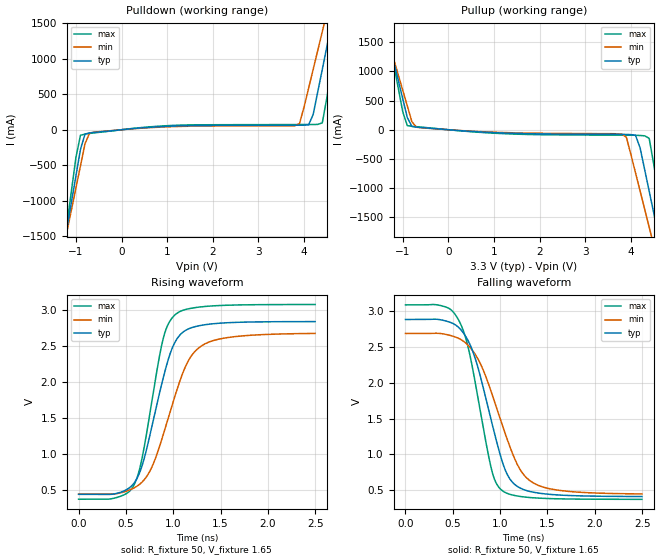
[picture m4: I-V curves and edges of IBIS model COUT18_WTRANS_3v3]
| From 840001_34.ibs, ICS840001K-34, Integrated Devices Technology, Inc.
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[Model] COUT18_WTRANS_3v3
Model_type   Output
Polarity   Non-Inverting
|   typ   min   max
C_comp   2pF   1.5pF   2.5pF
Vmeas = 1.65V
Rref = 50
Cref = 0
Vref = 1.65V
|   typ   min   max
[Voltage range]   3.3V   3.135V   3.465V
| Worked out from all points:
|   slope of the pulldown table from 0 to 0.495 V, typ, clamps not added: 17.2 ohm
|   slope of the pullup table from 0 to 0.495 V, typ, clamps not added: 17.5 ohm
|   rising waveform, R_fixture 50, V_fixture 1.65: 20-80 % time 269ps typ, 337ps min, 216ps max; typ from 0.443 V to 2.84 V
|   falling waveform, R_fixture 50, V_fixture 1.65: 20-80 % time 296ps typ, 367ps min, 235ps max; typ from 2.88 V to 0.414 V
[Pulldown]
|Voltage   I (typ)   I (min)   I (max)
-3.3V     -9.29A     -8.033A    -11.4A
-1.3V     -1.781A    -1.764A    -1.832A
-1.2V     -1.405A    -1.45A     -1.352A
-900mV    -277.4mA   -509.6mA   -77.59mA
-800mV    -60.69mA   -196.4mA   -61.25mA
-600mV    -38.28mA   -33.91mA   -44.11mA
3.9V      63.76mA    86.74mA    73.17mA
4.2V      215.8mA    852.4mA    74.01mA
4.4V      853.2mA    1.385A     97.44mA
4.6V      1.492A     1.918A     860.7mA
4.8V      2.133A     2.453A     1.678A
6.6V      8.005A     7.35A      9.166A
[Pullup]
|Voltage   I (typ)   I (min)   I (max)
-3.3V     7.952A     6.873A     9.764A
-1.4V     1.821A     1.753A     1.953A
-900mV    207mA      406.2mA    70.87mA
-700mV    45.36mA    43.45mA    52.59mA
3.8V      -79.73mA   -73.83mA   -93.19mA
3.9V      -80.98mA   -129.5mA   -93.43mA
4.1V      -95.21mA   -738mA     -95.04mA
4.3V      -681.6mA   -1.361A    -104.1mA
4.4V      -1.055A    -1.672A    -147.7mA
4.6V      -1.803A    -2.296A    -1.07A
4.8V      -2.551A    -2.921A    -2.024A
6.6V      -9.288A    -8.544A    -10.61A
[Ramp]
|   typ   min   max
dV/dt_r   1.921/0.415n   1.787/0.542n   2.166/0.338n
dV/dt_f   1.974/0.462n   1.788/0.58n   2.169/0.36n
R_load =   50.0000
[Rising Waveform]
R_fixture = 50
V_fixture = 1.65   |Vcc_typ
V_fixture_min = 1.5675 |Vcc_min
V_fixture_max = 1.7325 |Vcc_max
C_fixture = 0.0p
| Time   typ   min   max
0s        443.3mV    446.1mV    375.2mV
390.4ps   452mV      450.8mV    394.2mV
585.6ps   599.2mV    532.4mV    574.5mV
675.7ps   862.9mV    619.9mV    980.1mV
778.3ps   1.41V      835mV      1.772V
890.9ps   2.046V     1.259V     2.593V
1.026ns   2.576V     1.845V     2.946V
1.176ns   2.751V     2.338V     3.026V
1.364ns   2.805V     2.552V     3.057V
2.498ns   2.844V     2.679V     3.081V
[Falling Waveform]
R_fixture = 50
V_fixture = 1.65   |Vcc_typ
V_fixture_min = 1.5675 |Vcc_min
V_fixture_max = 1.7325 |Vcc_max
C_fixture = 0.0p
| Time   typ   min   max
0s        2.878V     2.683V     3.082V
405.4ps   2.865V     2.676V     3.06V
565.6ps   2.763V     2.613V     2.861V
645.6ps   2.622V     2.54V      2.576V
723.2ps   2.39V      2.42V      2.099V
910.9ps   1.448V     1.852V     781.2mV
1.016ns   927.2mV    1.435V     503mV
1.199ns   541.3mV    817.3mV    418mV
1.374ns   468.9mV    587mV      394.7mV
2.498ns   414.3mV    450.6mV    375.5mV
